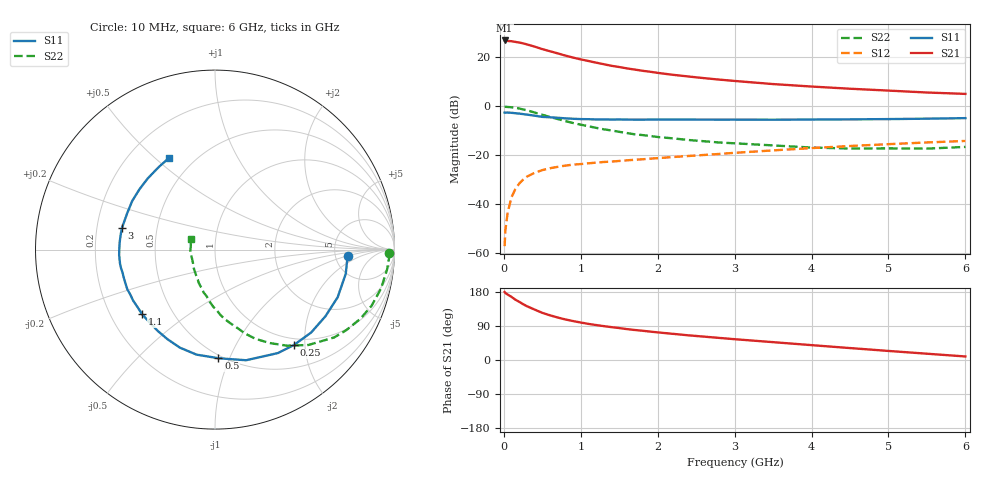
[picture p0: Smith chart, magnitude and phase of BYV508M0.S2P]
! SIEMENS Small Signal Semiconductors
! BFY420
! Si NPN RF SIEGET Grounded Emitter Transistor in MICRO-X
! VCE = 0.5 V  IC = 8 mA
! Common Emitter S-Parameters:  October  1996
# GHz  S  MA  R  50
!  f  S11  S21  S12  S22
! GHz  MAG  ANG  MAG  ANG  MAG  ANG  MAG  ANG
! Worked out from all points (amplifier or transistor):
!   36 points, 10 MHz to 6 GHz, reference 50 ohm
!   highest |S21| = 26.8 dB at 10 MHz (marker M1)
!   |S21| within 3 dB of that: start of sweep to 447.6 MHz
!   unconditionally stable (mu >= 1): 2.46 GHz to end of sweep
!   at 250 MHz: K = 0.17, MSG = 27.8 dB, |S12| = -30.0 dB
!   at 1.4 GHz: K = 0.73, MSG = 19.5 dB, |S12| = -22.6 dB
!   at 6 GHz: K = 1.15, MAG = 7.3 dB, |S12| = -14.2 dB
!   S11 on the Smith chart (normalised r, x): 10 MHz: 6.58, -0.98; 250 MHz: 0.88, -1.78; 500 MHz: 0.48, -0.91; 1.1 GHz: 0.33, -0.34; 3 GHz: 0.31, +0.10; 6 GHz: 0.37, +0.55
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0.01  0.7414 -2.6  21.89 179.4  0.0014 93.0  0.9677 -1.1
0.02  0.7388 -4.6  21.87 176.8  0.003 85.8  0.9714 -2.5
0.05  0.7408 -10.5  21.35 172.6  0.0068 85.0  0.9651 -6.6
0.1  0.7332 -21.2  21.13 166.6  0.014 80.6  0.9501 -13.2
0.15  0.7188 -31.1  20.45 159.1  0.0204 74.0  0.9269 -19.7
0.2  0.7074 -40.8  19.88 153.6  0.0265 71.1  0.8972 -25.4
0.25  0.6897 -50.5  19.08 147.3  0.0318 65.3  0.8591 -31.4
0.3  0.6746 -58.7  18.19 142.0  0.0366 62.7  0.8248 -36.4
0.4  0.6404 -74.3  16.39 133.0  0.0439 55.9  0.7438 -45.6
0.5  0.6055 -88.2  14.58 124.4  0.0497 50.9  0.6687 -53.2
0.6  0.5941 -100.0  13.2 117.9  0.0543 47.5  0.6028 -59.7
0.8  0.5652 -117.9  10.76 107.0  0.0615 42.2  0.4966 -70.3
0.9  0.5544 -124.9  9.79 102.7  0.0643 40.7  0.4539 -74.1
1.1  0.5431 -138.4  8.345 95.3  0.0685 38.6  0.3896 -82.2
1.3  0.5375 -147.9  7.169 89.4  0.0729 37.7  0.3378 -88.3
1.6  0.5331 -159.6  5.893 81.5  0.0787 36.9  0.2835 -97.1
2.2  0.5349 -176.7  4.358 69.0  0.092 35.8  0.2208 -111.2
3  0.5322 167.0  3.27 54.9  0.1119 34.0  0.1751 -127.6
3.5  0.5296 157.7  2.826 47.1  0.1256 31.9  0.1586 -137.8
4.5  0.5388 141.2  2.271 31.5  0.1544 25.4  0.1371 -159.5
5.5  0.5567 124.2  1.901 16.6  0.1823 17.2  0.1365 170.6
6  0.5709 116.9  1.782 9.3  0.1956 12.8  0.1479 157.0
